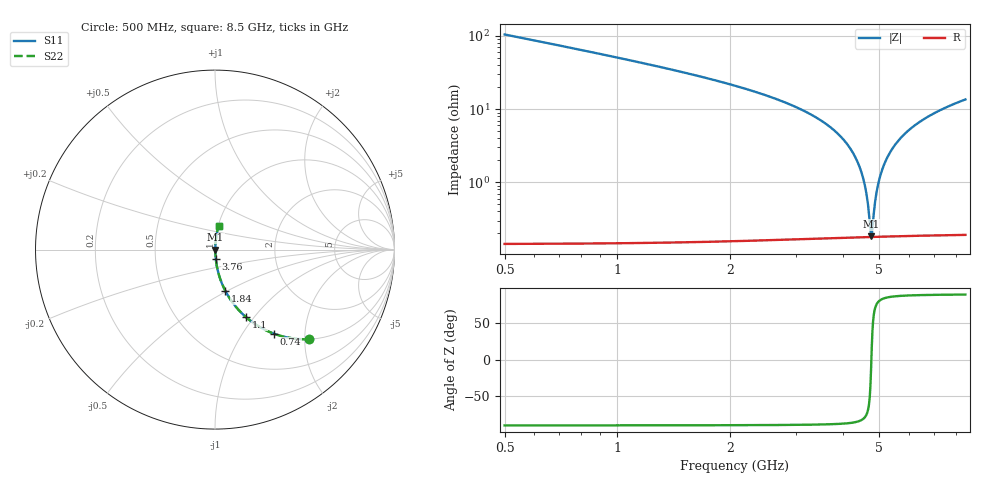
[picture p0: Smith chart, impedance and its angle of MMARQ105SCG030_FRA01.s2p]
! MMARQ105SCG030_FRA01  S-PARAMETER MODEL  ( General Type )
! Model Generated by TAIYO YUDEN Corporation (http://www.ty-top.com)
! Version 1.0
! TAIYO YUDEN Control No. 200326
! Copyright(c) 2020 TAIYO YUDEN CO.,LTD. All Rights Reserved.
! Product Description (link to TY-COMPAS)
! https://ds.yuden.co.jp/TYCOMPAS/or/detail?pn=MMARQ105SCG030BFRA01&u=M
! Products Name : Multilayer Ceramic Capacitors
! Characteristics :
!  Capacitance : 3 pF , Rated Voltage : 250V , TCC : CG / C0G
!  Case Size : 1.0 x 0.5 / 0.039 x 0.02 [mm/inch] , Thickness : 0.5 / 0.02 [mm/inch]
!  (Conditions: Temperature = 25 degC , DC Bias Current/Voltage = 0A / 0V)
! External Node Assignments :
!  1  o---| |---o  2
! GND o---------o GND
! Frequency Range : 500MHz  -  8.5GHz  [ 401 STEP ]
# MHz S RI R 50
! Freq[MHz].  S11 Real  S11 Imag  S21 Real  S21 Imag  S12 Real  S12 Imag  S22 Real  S22 Imag
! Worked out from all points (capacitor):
!   401 points, 500 MHz to 8.5 GHz, reference 50 ohm
!   read as one part in series: C = 3 pF near 540 MHz
!   lowest |Z| = 183 mohm at 4.76 GHz (marker M1)
!   series resonance near 4.768 GHz, so ESL is about 370 pH
!   S11 on the Smith chart (normalised r, x): 500 MHz: 1.00, -2.10; 740 MHz: 1.00, -1.40; 1.1 GHz: 1.00, -0.91; 1.84 GHz: 1.00, -0.49; 3.76 GHz: 1.00, -0.11; 8.5 GHz: 1.00, +0.27
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500  0.5246 -0.4987  0.4754 0.4987  0.4754 0.4987  0.5246 -0.4987
740  0.3294 -0.469  0.6706 0.469  0.6706 0.469  0.3294 -0.469
1100  0.1736 -0.3771  0.8264 0.3771  0.8264 0.3771  0.1736 -0.3771
1840  0.0581 -0.2309  0.9419 0.2309  0.9419 0.2309  0.0581 -0.2309
3180  0.0101 -0.0915  0.9899 0.0915  0.9899 0.0915  0.0101 -0.0915
3760  0.00455 -0.053  0.9955 0.053  0.9955 0.053  0.00455 -0.053
4200  0.00255 -0.0282  0.9974 0.0282  0.9974 0.0282  0.00255 -0.0282
4360  0.00216 -0.0199  0.9978 0.0199  0.9978 0.0199  0.00216 -0.0199
4500  0.00194 -0.0128  0.9981 0.0128  0.9981 0.0128  0.00194 -0.0128
4620  0.00183 -0.00699  0.9982 0.00699  0.9982 0.00699  0.00183 -0.00699
4660  0.00181 -0.00508  0.9982 0.00508  0.9982 0.00508  0.00181 -0.00508
4740  0.00179 -0.00131  0.9982 0.00131  0.9982 0.00131  0.00179 -0.00131
4760  0.00179 -0.000377  0.9982 0.000377  0.9982 0.000377  0.00179 -0.000377
4800  0.00179 0.00148  0.9982 -0.00148  0.9982 -0.00148  0.00179 0.00148
4880  0.00182 0.00514  0.9982 -0.00514  0.9982 -0.00514  0.00182 0.00514
4940  0.00186 0.00785  0.9981 -0.00785  0.9981 -0.00785  0.00186 0.00785
5120  0.00206 0.0158  0.9979 -0.0158  0.9979 -0.0158  0.00206 0.0158
5420  0.00263 0.0284  0.9974 -0.0284  0.9974 -0.0284  0.00263 0.0284
5840  0.00388 0.0451  0.9961 -0.0451  0.9961 -0.0451  0.00388 0.0451
6420  0.00632 0.0666  0.9937 -0.0666  0.9937 -0.0666  0.00632 0.0666
7180  0.0105 0.0924  0.9895 -0.0924  0.9895 -0.0924  0.0105 0.0924
8500  0.0199 0.1328  0.9801 -0.1328  0.9801 -0.1328  0.0199 0.1328
